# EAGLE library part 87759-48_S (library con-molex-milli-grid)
HEADER
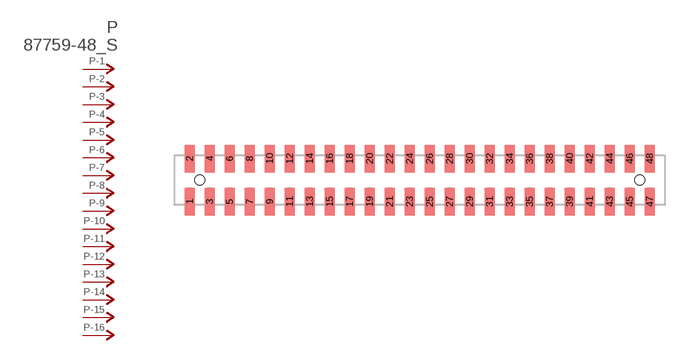
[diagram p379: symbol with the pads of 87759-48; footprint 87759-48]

Designator prefix P; gates -1=P-NV -2=P-N -3=P-N -4=P-N -5=P-N -6=P-N -7=P-N -8=P-N -9=P-N -10=P-N -11=P-N -12=P-N -13=P-N -14=P-N -15=P-N -16=P-N -17=P-N -18=P-N -19=P-N -20=P-N -21=P-N -22=P-N -23=P-N -24=P-N -25=P-N -26=P-N -27=P-N -28=P-N -29=P-N -30=P-N -31=P-N -32=P-N -33=P-N -34=P-N -35=P-N -36=P-N -37=P-N -38=P-N -39=P-N -40=P-N -41=P-N -42=P-N -43=P-N -44=P-N -45=P-N -46=P-N -47=P-N -48=P-N

## 87759-48_S  [87759-48]
1  -1:P  pas
2  -2:P  pas
3  -3:P  pas
4  -4:P  pas
5  -5:P  pas
6  -6:P  pas
7  -7:P  pas
8  -8:P  pas
9  -9:P  pas
10  -10:P  pas
11  -11:P  pas
12  -12:P  pas
13  -13:P  pas
14  -14:P  pas
15  -15:P  pas
16  -16:P  pas
17  -17:P  pas
18  -18:P  pas
19  -19:P  pas
20  -20:P  pas
21  -21:P  pas
22  -22:P  pas
23  -23:P  pas
24  -24:P  pas
25  -25:P  pas
26  -26:P  pas
27  -27:P  pas
28  -28:P  pas
29  -29:P  pas
30  -30:P  pas
31  -31:P  pas
32  -32:P  pas
33  -33:P  pas
34  -34:P  pas
35  -35:P  pas
36  -36:P  pas
37  -37:P  pas
38  -38:P  pas
39  -39:P  pas
40  -40:P  pas
41  -41:P  pas
42  -42:P  pas
43  -43:P  pas
44  -44:P  pas
45  -45:P  pas
46  -46:P  pas
47  -47:P  pas
48  -48:P  pas

## Footprint 87759-48 (pad centres in mm)
HEADER SMD Dual Row, Vertical
smd 1 x 2.75: 1 -23,-2.15; 2 -23,2.15; 3 -21,-2.15; 4 -21,2.15; 5 -19,-2.15; 6 -19,2.15; 7 -17,-2.15; 8 -17,2.15; 9 -15,-2.15; 10 -15,2.15; 11 -13,-2.15; 12 -13,2.15; 13 -11,-2.15; 14 -11,2.15; 15 -9,-2.15; 16 -9,2.15; 17 -7,-2.15; 18 -7,2.15; 19 -5,-2.15; 20 -5,2.15; 21 -3,-2.15; 22 -3,2.15; 23 -1,-2.15; 24 -1,2.15; 25 1,-2.15; 26 1,2.15; 27 3,-2.15; 28 3,2.15; 29 5,-2.15; 30 5,2.15; 31 7,-2.15; 32 7,2.15; 33 9,-2.15; 34 9,2.15; 35 11,-2.15; 36 11,2.15; 37 13,-2.15; 38 13,2.15; 39 15,-2.15; 40 15,2.15; 41 17,-2.15; 42 17,2.15; 43 19,-2.15; 44 19,2.15; 45 21,-2.15; 46 21,2.15; 47 23,-2.15; 48 23,2.15
hole 1 at -22,0
hole 1 at 22,0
